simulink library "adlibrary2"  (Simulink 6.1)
undefined symbols (not defined in the file or in its folder): adlibrary2, ADM, Bit, Black, Box, d2sram_config, DDR, ddr32_config, ddr32xp_config, Generation, II, Inactive, Location, Lower, SDRAM, Simulation, Subsystem, Width, xbsIndex_r3, XPL, XRC, XRM, zbt32_config, zbt64_config, zbtXRC4_config
libraries: xbsIndex_r3 x786
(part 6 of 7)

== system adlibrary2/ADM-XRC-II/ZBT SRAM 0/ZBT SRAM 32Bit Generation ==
  d : Inport  Port=1  LatchInput=off
  a : Inport  Port=2  LatchInput=off
  w : Inport  Port=3  LatchInput=off
  r : Inport  Port=4  LatchInput=off
  be : Inport  Port=5  LatchInput=off
  adlocb_in : Inport  Port=6  LatchInput=off
  Black Box : S-Function  FunctionName=xlblackbox2  Parameters=sfcn_mwsv__  mask(Xilinx Blackbox Block){init_code=zbt32_config, sim_method=Inactive, engine_block=, show_param=on, xl_area=[88, 129, 0, 35, 0, 0, 0], xl_use_area=on, adlocb_devid=0}
      mask prompts: init_code "Block Configuration M-Function"; sim_method "Simulation Mode"; engine_block "HDL Co-Simulator To Use  (specify helper block by name)"; show_param "---------------------- Show Implementation Parameters -----------------------------------------------------------------------------------"; xl_area "FPGA Area [Slices, FFs, BRAMs, LUTs, IOBs, Emb. Mults, TBUFs]"; xl_use_area "Use Area Above For Estimation"; adlocb_devid "ADLOCB DEV ID"
      mask help: Incorporates black box HDL and simulation model into a System Generator design. You must supply a Black Box with certain information about the HDL component you would like to bring into System Generator. This information is provided through a Matlab function. When "Simulation Mode" is set to "Inactive," you will typically want to provide a separate simulation model by using a Simulation Multiplexer. When "Simulation Mode" is set to "Use HDL Co-Simulation", you must include a ModelSim block in the design.
      mask init:
      | [designRoot, family, part, speed, package, simulinkPeriod, sysclkPeriod, dbl_ovrd, trimVbit] = xlSysgenSettings(gcb,0,0);
      | 
      | [bg,fg] = xlcmap('XBlock');
      | iPos = get_param(gcb,'Position');
      | iWidth=iPos(3)-iPos(1); iHeight=iPos(4)-iPos(2);
      | iCx=iWidth/2;
      | iCy=iHeight/2;
      | [logoX, logoY] = xlogo(iPos);
      | zstr='z'; zpstr='-1';
      | zstrx = iCx-3; if (zstrx<16) zstr='';zpstr=''; end
      | zstry = iCy;
      | 
      | precision0 = 1;
      | latency = 0;
      | dblOvrd = 0;
      | 
      | mdlPath = xlGetMdlDir(bdroot);
      | 
      | refBlk = get_param(gcb,'referenceBlock');
      | if (isempty(refBlk) | strncmp(refBlk,'xbsIndex',8))
      | 	srcPath = mdlPath;
      | else
      | 	srcPath = xlPathToReference;
      | 	if (isempty(srcPath))
      | 		srcPath = mdlPath;
      | 	end
      | end
      | 
      | if (sim_method==2)
      | 	validEngineBlock = 0;
      | 	try
      | 	  engineBlock = xlBlockNameRelPath(get_param(gcb,'Parent'),engine_block);
      | 	catch
      | 	  engineBlock = '//';
      | 	end
      | 	try 
      | 	  engineWorkDir = get_param(engineBlock,'dir');
      | 	  validEngineBlock = 1;
      | 	catch
      | 	end
      | end
      | 
      | % just pass everything to s-function
      | sfcn_mwsv__ = get_param(gcb, 'MaskWSVariables');
      | 
      | plabel = xlbbPortLabelStruct(gcb,init_code,mdlPath);
  Constant : Constant  Value=0
  Convert : xbsIndex_r3/Convert  arith_type=Unsigned  n_bits=34  bin_pt=0  quantization=Truncate  overflow=Wrap  latency=0  explicit_period=on  period=1  dbl_ovrd=off  show_param=off  inserted_by_tool=off  pipeline=off
  Terminator{,1..3} (4 alike) : Terminator
  ra0 : xbsIndex_r3/Gateway Out  output_type=Double  nbits=8  bin_pt=6  arith_type=Boolean  quantization=Truncate  overflow=Wrap  hdl_port=on  timing_constraint=None  locs_specified=off  LOCs={}  needs_fixed_name=off  show_param=off
  rc0 : xbsIndex_r3/Gateway Out  output_type=Double  nbits=8  bin_pt=6  arith_type=Boolean  quantization=Truncate  overflow=Wrap  hdl_port=on  timing_constraint=None  locs_specified=off  LOCs={}  needs_fixed_name=off  show_param=off
  rd0_i : xbsIndex_r3/Gateway In  arith_type=Unsigned  n_bits=32  bin_pt=0  quantization=Truncate  overflow=Wrap  period=1  timing_constraint=None  locs_specified=off  LOCs={}  needs_fixed_name=off  dbl_ovrd=off  show_param=off
  rd0_o : xbsIndex_r3/Gateway Out  output_type=Double  nbits=8  bin_pt=6  arith_type=Boolean  quantization=Truncate  overflow=Wrap  hdl_port=on  timing_constraint=None  locs_specified=off  LOCs={}  needs_fixed_name=off  show_param=off
  rd0_t : xbsIndex_r3/Gateway Out  output_type=Double  nbits=8  bin_pt=6  arith_type=Boolean  quantization=Truncate  overflow=Wrap  hdl_port=on  timing_constraint=None  locs_specified=off  LOCs={}  needs_fixed_name=off  show_param=off
  q : Outport
  qv : Outport  Port=2
  adlocb_out : Outport  Port=3
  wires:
  Black Box/6 -> rc0/1
  Black Box/5 -> ra0/1
  Black Box/4 -> rd0_t/1
  Black Box/3 -> rd0_o/1
  r/1 -> Black Box/4
  w/1 -> Black Box/3
  a/1 -> Black Box/2
  rc0/1 -> Terminator3/1
  ra0/1 -> Terminator2/1
  rd0_t/1 -> Terminator1/1
  rd0_o/1 -> Terminator/1
  Constant/1 -> rd0_i/1
  Black Box/2 -> qv/1
  Black Box/1 -> q/1
  d/1 -> Black Box/1
  rd0_i/1 -> Black Box/6
  be/1 -> Black Box/5
  adlocb_in/1 -> Black Box/7
  Black Box/7 -> Convert/1
  Convert/1 -> adlocb_out/1

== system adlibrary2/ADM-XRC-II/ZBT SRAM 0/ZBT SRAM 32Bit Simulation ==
  d : Inport  Port=1  LatchInput=off
  a : Inport  Port=2  LatchInput=off
  w : Inport  Port=3  LatchInput=off
  r : Inport  Port=4  LatchInput=off
  be : Inport  Port=5  LatchInput=off
  Disregard Subsystem : xbsIndex_r3/Disregard Subsystem  Tag=discardX
  Gateway In6 : xbsIndex_r3/Gateway In  arith_type=Boolean  n_bits=1  bin_pt=0  quantization=Truncate  overflow=Wrap  period=1  timing_constraint=None  locs_specified=off  LOCs={}  needs_fixed_name=off  dbl_ovrd=on  show_param=off
  Gateway In7 : xbsIndex_r3/Gateway In  arith_type=Unsigned  n_bits=32  bin_pt=0  quantization=Truncate  overflow=Wrap  period=1  timing_constraint=None  locs_specified=off  LOCs={}  needs_fixed_name=off  dbl_ovrd=on  show_param=off
  Gateway Out{,1..4} (5 alike) : xbsIndex_r3/Gateway Out  output_type=Double  nbits=8  bin_pt=6  arith_type=Boolean  quantization=Truncate  overflow=Wrap  hdl_port=off  timing_constraint=None  locs_specified=off  LOCs={}  needs_fixed_name=off  show_param=off
  S-Function : S-Function  FunctionName=zbt32  Parameters=0
  q : Outport
  qv : Outport  Port=2
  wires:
  S-Function/2 -> Gateway In6/1
  Gateway In7/1 -> q/1
  Gateway In6/1 -> qv/1
  Gateway Out3/1 -> S-Function/4
  Gateway Out2/1 -> S-Function/3
  Gateway Out1/1 -> S-Function/2
  Gateway Out/1 -> S-Function/1
  S-Function/1 -> Gateway In7/1
  r/1 -> Gateway Out3/1
  w/1 -> Gateway Out2/1
  a/1 -> Gateway Out1/1
  d/1 -> Gateway Out/1
  Gateway Out4/1 -> S-Function/5
  be/1 -> Gateway Out4/1

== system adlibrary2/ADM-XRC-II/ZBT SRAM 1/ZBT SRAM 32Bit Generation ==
  d : Inport  Port=1  LatchInput=off
  a : Inport  Port=2  LatchInput=off
  w : Inport  Port=3  LatchInput=off
  r : Inport  Port=4  LatchInput=off
  be : Inport  Port=5  LatchInput=off
  adlocb_in : Inport  Port=6  LatchInput=off
  Black Box : S-Function  FunctionName=xlblackbox2  Parameters=sfcn_mwsv__  mask(Xilinx Blackbox Block){init_code=zbt32_config, sim_method=Inactive, engine_block=, show_param=on, xl_area=[88, 129, 0, 35, 0, 0, 0], xl_use_area=on, adlocb_devid=1}
      mask prompts: init_code "Block Configuration M-Function"; sim_method "Simulation Mode"; engine_block "HDL Co-Simulator To Use  (specify helper block by name)"; show_param "---------------------- Show Implementation Parameters -----------------------------------------------------------------------------------"; xl_area "FPGA Area [Slices, FFs, BRAMs, LUTs, IOBs, Emb. Mults, TBUFs]"; xl_use_area "Use Area Above For Estimation"; adlocb_devid "ADLOCB DEV ID"
      mask help: Incorporates black box HDL and simulation model into a System Generator design. You must supply a Black Box with certain information about the HDL component you would like to bring into System Generator. This information is provided through a Matlab function. When "Simulation Mode" is set to "Inactive," you will typically want to provide a separate simulation model by using a Simulation Multiplexer. When "Simulation Mode" is set to "Use HDL Co-Simulation", you must include a ModelSim block in the design.
      mask init:
      | [designRoot, family, part, speed, package, simulinkPeriod, sysclkPeriod, dbl_ovrd, trimVbit] = xlSysgenSettings(gcb,0,0);
      | 
      | [bg,fg] = xlcmap('XBlock');
      | iPos = get_param(gcb,'Position');
      | iWidth=iPos(3)-iPos(1); iHeight=iPos(4)-iPos(2);
      | iCx=iWidth/2;
      | iCy=iHeight/2;
      | [logoX, logoY] = xlogo(iPos);
      | zstr='z'; zpstr='-1';
      | zstrx = iCx-3; if (zstrx<16) zstr='';zpstr=''; end
      | zstry = iCy;
      | 
      | precision0 = 1;
      | latency = 0;
      | dblOvrd = 0;
      | 
      | mdlPath = xlGetMdlDir(bdroot);
      | 
      | refBlk = get_param(gcb,'referenceBlock');
      | if (isempty(refBlk) | strncmp(refBlk,'xbsIndex',8))
      | 	srcPath = mdlPath;
      | else
      | 	srcPath = xlPathToReference;
      | 	if (isempty(srcPath))
      | 		srcPath = mdlPath;
      | 	end
      | end
      | 
      | if (sim_method==2)
      | 	validEngineBlock = 0;
      | 	try
      | 	  engineBlock = xlBlockNameRelPath(get_param(gcb,'Parent'),engine_block);
      | 	catch
      | 	  engineBlock = '//';
      | 	end
      | 	try 
      | 	  engineWorkDir = get_param(engineBlock,'dir');
      | 	  validEngineBlock = 1;
      | 	catch
      | 	end
      | end
      | 
      | % just pass everything to s-function
      | sfcn_mwsv__ = get_param(gcb, 'MaskWSVariables');
      | adlocb_devid = 1;
      | plabel = xlbbPortLabelStruct(gcb,init_code,mdlPath);
  Constant : Constant  Value=0
  Terminator{,1..3} (4 alike) : Terminator
  ra1 : xbsIndex_r3/Gateway Out  output_type=Double  nbits=8  bin_pt=6  arith_type=Boolean  quantization=Truncate  overflow=Wrap  hdl_port=on  timing_constraint=None  locs_specified=off  LOCs={}  needs_fixed_name=off  show_param=off
  rc1 : xbsIndex_r3/Gateway Out  output_type=Double  nbits=8  bin_pt=6  arith_type=Boolean  quantization=Truncate  overflow=Wrap  hdl_port=on  timing_constraint=None  locs_specified=off  LOCs={}  needs_fixed_name=off  show_param=off
  rd1_i : xbsIndex_r3/Gateway In  arith_type=Unsigned  n_bits=32  bin_pt=0  quantization=Truncate  overflow=Wrap  period=1  timing_constraint=None  locs_specified=off  LOCs={}  needs_fixed_name=off  dbl_ovrd=off  show_param=off
  rd1_o : xbsIndex_r3/Gateway Out  output_type=Double  nbits=8  bin_pt=6  arith_type=Boolean  quantization=Truncate  overflow=Wrap  hdl_port=on  timing_constraint=None  locs_specified=off  LOCs={}  needs_fixed_name=off  show_param=off
  rd1_t : xbsIndex_r3/Gateway Out  output_type=Double  nbits=8  bin_pt=6  arith_type=Boolean  quantization=Truncate  overflow=Wrap  hdl_port=on  timing_constraint=None  locs_specified=off  LOCs={}  needs_fixed_name=off  show_param=off
  q : Outport
  qv : Outport  Port=2
  adlocb_out : Outport  Port=3
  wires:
  Black Box/7 -> adlocb_out/1
  adlocb_in/1 -> Black Box/7
  be/1 -> Black Box/5
  rd1_i/1 -> Black Box/6
  d/1 -> Black Box/1
  Black Box/1 -> q/1
  Black Box/2 -> qv/1
  Constant/1 -> rd1_i/1
  rd1_o/1 -> Terminator/1
  rd1_t/1 -> Terminator1/1
  ra1/1 -> Terminator2/1
  rc1/1 -> Terminator3/1
  a/1 -> Black Box/2
  w/1 -> Black Box/3
  r/1 -> Black Box/4
  Black Box/3 -> rd1_o/1
  Black Box/4 -> rd1_t/1
  Black Box/5 -> ra1/1
  Black Box/6 -> rc1/1

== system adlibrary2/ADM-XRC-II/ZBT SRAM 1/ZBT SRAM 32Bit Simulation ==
  d : Inport  Port=1  LatchInput=off
  a : Inport  Port=2  LatchInput=off
  w : Inport  Port=3  LatchInput=off
  r : Inport  Port=4  LatchInput=off
  be : Inport  Port=5  LatchInput=off
  Disregard Subsystem : xbsIndex_r3/Disregard Subsystem  Tag=discardX
  Gateway In6 : xbsIndex_r3/Gateway In  arith_type=Boolean  n_bits=1  bin_pt=0  quantization=Truncate  overflow=Wrap  period=1  timing_constraint=None  locs_specified=off  LOCs={}  needs_fixed_name=off  dbl_ovrd=on  show_param=off
  Gateway In7 : xbsIndex_r3/Gateway In  arith_type=Unsigned  n_bits=32  bin_pt=0  quantization=Truncate  overflow=Wrap  period=1  timing_constraint=None  locs_specified=off  LOCs={}  needs_fixed_name=off  dbl_ovrd=on  show_param=off
  Gateway Out{,1..4} (5 alike) : xbsIndex_r3/Gateway Out  output_type=Double  nbits=8  bin_pt=6  arith_type=Boolean  quantization=Truncate  overflow=Wrap  hdl_port=off  timing_constraint=None  locs_specified=off  LOCs={}  needs_fixed_name=off  show_param=off
  S-Function : S-Function  FunctionName=zbt32  Parameters=1
  q : Outport
  qv : Outport  Port=2
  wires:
  be/1 -> Gateway Out4/1
  Gateway Out4/1 -> S-Function/5
  d/1 -> Gateway Out/1
  a/1 -> Gateway Out1/1
  w/1 -> Gateway Out2/1
  r/1 -> Gateway Out3/1
  S-Function/1 -> Gateway In7/1
  Gateway Out/1 -> S-Function/1
  Gateway Out1/1 -> S-Function/2
  Gateway Out2/1 -> S-Function/3
  Gateway Out3/1 -> S-Function/4
  Gateway In6/1 -> qv/1
  Gateway In7/1 -> q/1
  S-Function/2 -> Gateway In6/1

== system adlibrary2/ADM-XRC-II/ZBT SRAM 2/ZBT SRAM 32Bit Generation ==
  d : Inport  Port=1  LatchInput=off
  a : Inport  Port=2  LatchInput=off
  w : Inport  Port=3  LatchInput=off
  r : Inport  Port=4  LatchInput=off
  be : Inport  Port=5  LatchInput=off
  adlocb_in : Inport  Port=6  LatchInput=off
  Black Box : S-Function  FunctionName=xlblackbox2  Parameters=sfcn_mwsv__  mask(Xilinx Blackbox Block){init_code=zbt32_config, sim_method=Inactive, engine_block=, show_param=on, xl_area=[88, 129, 0, 35, 0, 0, 0], xl_use_area=on, adlocb_devid=2}
      mask prompts: init_code "Block Configuration M-Function"; sim_method "Simulation Mode"; engine_block "HDL Co-Simulator To Use  (specify helper block by name)"; show_param "---------------------- Show Implementation Parameters -----------------------------------------------------------------------------------"; xl_area "FPGA Area [Slices, FFs, BRAMs, LUTs, IOBs, Emb. Mults, TBUFs]"; xl_use_area "Use Area Above For Estimation"; adlocb_devid "ADLOCB DEV ID"
      mask help: Incorporates black box HDL and simulation model into a System Generator design. You must supply a Black Box with certain information about the HDL component you would like to bring into System Generator. This information is provided through a Matlab function. When "Simulation Mode" is set to "Inactive," you will typically want to provide a separate simulation model by using a Simulation Multiplexer. When "Simulation Mode" is set to "Use HDL Co-Simulation", you must include a ModelSim block in the design.
      mask init:
      | [designRoot, family, part, speed, package, simulinkPeriod, sysclkPeriod, dbl_ovrd, trimVbit] = xlSysgenSettings(gcb,0,0);
      | 
      | [bg,fg] = xlcmap('XBlock');
      | iPos = get_param(gcb,'Position');
      | iWidth=iPos(3)-iPos(1); iHeight=iPos(4)-iPos(2);
      | iCx=iWidth/2;
      | iCy=iHeight/2;
      | [logoX, logoY] = xlogo(iPos);
      | zstr='z'; zpstr='-1';
      | zstrx = iCx-3; if (zstrx<16) zstr='';zpstr=''; end
      | zstry = iCy;
      | 
      | precision0 = 1;
      | latency = 0;
      | dblOvrd = 0;
      | 
      | mdlPath = xlGetMdlDir(bdroot);
      | 
      | refBlk = get_param(gcb,'referenceBlock');
      | if (isempty(refBlk) | strncmp(refBlk,'xbsIndex',8))
      | 	srcPath = mdlPath;
      | else
      | 	srcPath = xlPathToReference;
      | 	if (isempty(srcPath))
      | 		srcPath = mdlPath;
      | 	end
      | end
      | 
      | if (sim_method==2)
      | 	validEngineBlock = 0;
      | 	try
      | 	  engineBlock = xlBlockNameRelPath(get_param(gcb,'Parent'),engine_block);
      | 	catch
      | 	  engineBlock = '//';
      | 	end
      | 	try 
      | 	  engineWorkDir = get_param(engineBlock,'dir');
      | 	  validEngineBlock = 1;
      | 	catch
      | 	end
      | end
      | 
      | % just pass everything to s-function
      | sfcn_mwsv__ = get_param(gcb, 'MaskWSVariables');
      | 
      | plabel = xlbbPortLabelStruct(gcb,init_code,mdlPath);
  Constant : Constant  Value=0
  Terminator{,1..3} (4 alike) : Terminator
  ra2 : xbsIndex_r3/Gateway Out  output_type=Double  nbits=8  bin_pt=6  arith_type=Boolean  quantization=Truncate  overflow=Wrap  hdl_port=on  timing_constraint=None  locs_specified=off  LOCs={}  needs_fixed_name=off  show_param=off
  rc2 : xbsIndex_r3/Gateway Out  output_type=Double  nbits=8  bin_pt=6  arith_type=Boolean  quantization=Truncate  overflow=Wrap  hdl_port=on  timing_constraint=None  locs_specified=off  LOCs={}  needs_fixed_name=off  show_param=off
  rd2_i : xbsIndex_r3/Gateway In  arith_type=Unsigned  n_bits=32  bin_pt=0  quantization=Truncate  overflow=Wrap  period=1  timing_constraint=None  locs_specified=off  LOCs={}  needs_fixed_name=off  dbl_ovrd=off  show_param=off
  rd2_o : xbsIndex_r3/Gateway Out  output_type=Double  nbits=8  bin_pt=6  arith_type=Boolean  quantization=Truncate  overflow=Wrap  hdl_port=on  timing_constraint=None  locs_specified=off  LOCs={}  needs_fixed_name=off  show_param=off
  rd2_t : xbsIndex_r3/Gateway Out  output_type=Double  nbits=8  bin_pt=6  arith_type=Boolean  quantization=Truncate  overflow=Wrap  hdl_port=on  timing_constraint=None  locs_specified=off  LOCs={}  needs_fixed_name=off  show_param=off
  q : Outport
  qv : Outport  Port=2
  adlocb_out : Outport  Port=3
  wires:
  Black Box/7 -> adlocb_out/1
  adlocb_in/1 -> Black Box/7
  be/1 -> Black Box/5
  rd2_i/1 -> Black Box/6
  d/1 -> Black Box/1
  Black Box/1 -> q/1
  Black Box/2 -> qv/1
  Constant/1 -> rd2_i/1
  rd2_o/1 -> Terminator/1
  rd2_t/1 -> Terminator1/1
  ra2/1 -> Terminator2/1
  rc2/1 -> Terminator3/1
  a/1 -> Black Box/2
  w/1 -> Black Box/3
  r/1 -> Black Box/4
  Black Box/3 -> rd2_o/1
  Black Box/4 -> rd2_t/1
  Black Box/5 -> ra2/1
  Black Box/6 -> rc2/1

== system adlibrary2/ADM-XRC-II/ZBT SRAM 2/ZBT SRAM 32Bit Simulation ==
  d : Inport  Port=1  LatchInput=off
  a : Inport  Port=2  LatchInput=off
  w : Inport  Port=3  LatchInput=off
  r : Inport  Port=4  LatchInput=off
  be : Inport  Port=5  LatchInput=off
  Disregard Subsystem : xbsIndex_r3/Disregard Subsystem  Tag=discardX
  Gateway In6 : xbsIndex_r3/Gateway In  arith_type=Boolean  n_bits=1  bin_pt=0  quantization=Truncate  overflow=Wrap  period=1  timing_constraint=None  locs_specified=off  LOCs={}  needs_fixed_name=off  dbl_ovrd=on  show_param=off
  Gateway In7 : xbsIndex_r3/Gateway In  arith_type=Unsigned  n_bits=32  bin_pt=0  quantization=Truncate  overflow=Wrap  period=1  timing_constraint=None  locs_specified=off  LOCs={}  needs_fixed_name=off  dbl_ovrd=on  show_param=off
  Gateway Out{,1..4} (5 alike) : xbsIndex_r3/Gateway Out  output_type=Double  nbits=8  bin_pt=6  arith_type=Boolean  quantization=Truncate  overflow=Wrap  hdl_port=off  timing_constraint=None  locs_specified=off  LOCs={}  needs_fixed_name=off  show_param=off
  S-Function : S-Function  FunctionName=zbt32  Parameters=2
  q : Outport
  qv : Outport  Port=2
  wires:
  be/1 -> Gateway Out4/1
  Gateway Out4/1 -> S-Function/5
  d/1 -> Gateway Out/1
  a/1 -> Gateway Out1/1
  w/1 -> Gateway Out2/1
  r/1 -> Gateway Out3/1
  S-Function/1 -> Gateway In7/1
  Gateway Out/1 -> S-Function/1
  Gateway Out1/1 -> S-Function/2
  Gateway Out2/1 -> S-Function/3
  Gateway Out3/1 -> S-Function/4
  Gateway In6/1 -> qv/1
  Gateway In7/1 -> q/1
  S-Function/2 -> Gateway In6/1

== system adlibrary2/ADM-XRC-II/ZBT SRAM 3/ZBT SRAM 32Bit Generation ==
  d : Inport  Port=1  LatchInput=off
  a : Inport  Port=2  LatchInput=off
  w : Inport  Port=3  LatchInput=off
  r : Inport  Port=4  LatchInput=off
  be : Inport  Port=5  LatchInput=off
  adlocb_in : Inport  Port=6  LatchInput=off
  Black Box : S-Function  FunctionName=xlblackbox2  Parameters=sfcn_mwsv__  mask(Xilinx Blackbox Block){init_code=zbt32_config, sim_method=Inactive, engine_block=, show_param=on, xl_area=[88, 129, 0, 35, 0, 0, 0], xl_use_area=on, adlocb_devid=3}
      mask prompts: init_code "Block Configuration M-Function"; sim_method "Simulation Mode"; engine_block "HDL Co-Simulator To Use  (specify helper block by name)"; show_param "---------------------- Show Implementation Parameters -----------------------------------------------------------------------------------"; xl_area "FPGA Area [Slices, FFs, BRAMs, LUTs, IOBs, Emb. Mults, TBUFs]"; xl_use_area "Use Area Above For Estimation"; adlocb_devid "ADLOCB DEV ID"
      mask help: Incorporates black box HDL and simulation model into a System Generator design. You must supply a Black Box with certain information about the HDL component you would like to bring into System Generator. This information is provided through a Matlab function. When "Simulation Mode" is set to "Inactive," you will typically want to provide a separate simulation model by using a Simulation Multiplexer. When "Simulation Mode" is set to "Use HDL Co-Simulation", you must include a ModelSim block in the design.
      mask init:
      | [designRoot, family, part, speed, package, simulinkPeriod, sysclkPeriod, dbl_ovrd, trimVbit] = xlSysgenSettings(gcb,0,0);
      | 
      | [bg,fg] = xlcmap('XBlock');
      | iPos = get_param(gcb,'Position');
      | iWidth=iPos(3)-iPos(1); iHeight=iPos(4)-iPos(2);
      | iCx=iWidth/2;
      | iCy=iHeight/2;
      | [logoX, logoY] = xlogo(iPos);
      | zstr='z'; zpstr='-1';
      | zstrx = iCx-3; if (zstrx<16) zstr='';zpstr=''; end
      | zstry = iCy;
      | 
      | precision0 = 1;
      | latency = 0;
      | dblOvrd = 0;
      | 
      | mdlPath = xlGetMdlDir(bdroot);
      | 
      | refBlk = get_param(gcb,'referenceBlock');
      | if (isempty(refBlk) | strncmp(refBlk,'xbsIndex',8))
      | 	srcPath = mdlPath;
      | else
      | 	srcPath = xlPathToReference;
      | 	if (isempty(srcPath))
      | 		srcPath = mdlPath;
      | 	end
      | end
      | 
      | if (sim_method==2)
      | 	validEngineBlock = 0;
      | 	try
      | 	  engineBlock = xlBlockNameRelPath(get_param(gcb,'Parent'),engine_block);
      | 	catch
      | 	  engineBlock = '//';
      | 	end
      | 	try 
      | 	  engineWorkDir = get_param(engineBlock,'dir');
      | 	  validEngineBlock = 1;
      | 	catch
      | 	end
      | end
      | 
      | % just pass everything to s-function
      | sfcn_mwsv__ = get_param(gcb, 'MaskWSVariables');
      | adlocb_devid = 1;
      | plabel = xlbbPortLabelStruct(gcb,init_code,mdlPath);
  Constant : Constant  Value=0
  Terminator{,1..3} (4 alike) : Terminator
  ra3 : xbsIndex_r3/Gateway Out  output_type=Double  nbits=8  bin_pt=6  arith_type=Boolean  quantization=Truncate  overflow=Wrap  hdl_port=on  timing_constraint=None  locs_specified=off  LOCs={}  needs_fixed_name=off  show_param=off
  rc3 : xbsIndex_r3/Gateway Out  output_type=Double  nbits=8  bin_pt=6  arith_type=Boolean  quantization=Truncate  overflow=Wrap  hdl_port=on  timing_constraint=None  locs_specified=off  LOCs={}  needs_fixed_name=off  show_param=off
  rd3_i : xbsIndex_r3/Gateway In  arith_type=Unsigned  n_bits=32  bin_pt=0  quantization=Truncate  overflow=Wrap  period=1  timing_constraint=None  locs_specified=off  LOCs={}  needs_fixed_name=off  dbl_ovrd=off  show_param=off
  rd3_o : xbsIndex_r3/Gateway Out  output_type=Double  nbits=8  bin_pt=6  arith_type=Boolean  quantization=Truncate  overflow=Wrap  hdl_port=on  timing_constraint=None  locs_specified=off  LOCs={}  needs_fixed_name=off  show_param=off
  rd3_t : xbsIndex_r3/Gateway Out  output_type=Double  nbits=8  bin_pt=6  arith_type=Boolean  quantization=Truncate  overflow=Wrap  hdl_port=on  timing_constraint=None  locs_specified=off  LOCs={}  needs_fixed_name=off  show_param=off
  q : Outport
  qv : Outport  Port=2
  adlocb_out : Outport  Port=3
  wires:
  Black Box/6 -> rc3/1
  Black Box/5 -> ra3/1
  Black Box/4 -> rd3_t/1
  Black Box/3 -> rd3_o/1
  r/1 -> Black Box/4
  w/1 -> Black Box/3
  a/1 -> Black Box/2
  rc3/1 -> Terminator3/1
  ra3/1 -> Terminator2/1
  rd3_t/1 -> Terminator1/1
  rd3_o/1 -> Terminator/1
  Constant/1 -> rd3_i/1
  Black Box/2 -> qv/1
  Black Box/1 -> q/1
  d/1 -> Black Box/1
  rd3_i/1 -> Black Box/6
  be/1 -> Black Box/5
  adlocb_in/1 -> Black Box/7
  Black Box/7 -> adlocb_out/1

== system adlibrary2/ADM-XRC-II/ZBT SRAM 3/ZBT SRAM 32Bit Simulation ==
  d : Inport  Port=1  LatchInput=off
  a : Inport  Port=2  LatchInput=off
  w : Inport  Port=3  LatchInput=off
  r : Inport  Port=4  LatchInput=off
  be : Inport  Port=5  LatchInput=off
  Disregard Subsystem : xbsIndex_r3/Disregard Subsystem  Tag=discardX
  Gateway In6 : xbsIndex_r3/Gateway In  arith_type=Boolean  n_bits=1  bin_pt=0  quantization=Truncate  overflow=Wrap  period=1  timing_constraint=None  locs_specified=off  LOCs={}  needs_fixed_name=off  dbl_ovrd=on  show_param=off
  Gateway In7 : xbsIndex_r3/Gateway In  arith_type=Unsigned  n_bits=32  bin_pt=0  quantization=Truncate  overflow=Wrap  period=1  timing_constraint=None  locs_specified=off  LOCs={}  needs_fixed_name=off  dbl_ovrd=on  show_param=off
  Gateway Out{,1..4} (5 alike) : xbsIndex_r3/Gateway Out  output_type=Double  nbits=8  bin_pt=6  arith_type=Boolean  quantization=Truncate  overflow=Wrap  hdl_port=off  timing_constraint=None  locs_specified=off  LOCs={}  needs_fixed_name=off  show_param=off
  S-Function : S-Function  FunctionName=zbt32  Parameters=3
  q : Outport
  qv : Outport  Port=2
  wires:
  S-Function/2 -> Gateway In6/1
  Gateway In7/1 -> q/1
  Gateway In6/1 -> qv/1
  Gateway Out3/1 -> S-Function/4
  Gateway Out2/1 -> S-Function/3
  Gateway Out1/1 -> S-Function/2
  Gateway Out/1 -> S-Function/1
  S-Function/1 -> Gateway In7/1
  r/1 -> Gateway Out3/1
  w/1 -> Gateway Out2/1
  a/1 -> Gateway Out1/1
  d/1 -> Gateway Out/1
  Gateway Out4/1 -> S-Function/5
  be/1 -> Gateway Out4/1

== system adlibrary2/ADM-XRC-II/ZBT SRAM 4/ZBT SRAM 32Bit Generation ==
  d : Inport  Port=1  LatchInput=off
  a : Inport  Port=2  LatchInput=off
  w : Inport  Port=3  LatchInput=off
  r : Inport  Port=4  LatchInput=off
  be : Inport  Port=5  LatchInput=off
  adlocb_in : Inport  Port=6  LatchInput=off
  Black Box : S-Function  FunctionName=xlblackbox2  Parameters=sfcn_mwsv__  mask(Xilinx Blackbox Block){init_code=zbt32_config, sim_method=Inactive, engine_block=, show_param=on, xl_area=[88, 129, 0, 35, 0, 0, 0], xl_use_area=on, adlocb_devid=4}
      mask prompts: init_code "Block Configuration M-Function"; sim_method "Simulation Mode"; engine_block "HDL Co-Simulator To Use  (specify helper block by name)"; show_param "---------------------- Show Implementation Parameters -----------------------------------------------------------------------------------"; xl_area "FPGA Area [Slices, FFs, BRAMs, LUTs, IOBs, Emb. Mults, TBUFs]"; xl_use_area "Use Area Above For Estimation"; adlocb_devid "ADLOCB DEV ID"
      mask help: Incorporates black box HDL and simulation model into a System Generator design. You must supply a Black Box with certain information about the HDL component you would like to bring into System Generator. This information is provided through a Matlab function. When "Simulation Mode" is set to "Inactive," you will typically want to provide a separate simulation model by using a Simulation Multiplexer. When "Simulation Mode" is set to "Use HDL Co-Simulation", you must include a ModelSim block in the design.
      mask init:
      | [designRoot, family, part, speed, package, simulinkPeriod, sysclkPeriod, dbl_ovrd, trimVbit] = xlSysgenSettings(gcb,0,0);
      | 
      | [bg,fg] = xlcmap('XBlock');
      | iPos = get_param(gcb,'Position');
      | iWidth=iPos(3)-iPos(1); iHeight=iPos(4)-iPos(2);
      | iCx=iWidth/2;
      | iCy=iHeight/2;
      | [logoX, logoY] = xlogo(iPos);
      | zstr='z'; zpstr='-1';
      | zstrx = iCx-3; if (zstrx<16) zstr='';zpstr=''; end
      | zstry = iCy;
      | 
      | precision0 = 1;
      | latency = 0;
      | dblOvrd = 0;
      | 
      | mdlPath = xlGetMdlDir(bdroot);
      | 
      | refBlk = get_param(gcb,'referenceBlock');
      | if (isempty(refBlk) | strncmp(refBlk,'xbsIndex',8))
      | 	srcPath = mdlPath;
      | else
      | 	srcPath = xlPathToReference;
      | 	if (isempty(srcPath))
      | 		srcPath = mdlPath;
      | 	end
      | end
      | 
      | if (sim_method==2)
      | 	validEngineBlock = 0;
      | 	try
      | 	  engineBlock = xlBlockNameRelPath(get_param(gcb,'Parent'),engine_block);
      | 	catch
      | 	  engineBlock = '//';
      | 	end
      | 	try 
      | 	  engineWorkDir = get_param(engineBlock,'dir');
      | 	  validEngineBlock = 1;
      | 	catch
      | 	end
      | end
      | 
      | % just pass everything to s-function
      | sfcn_mwsv__ = get_param(gcb, 'MaskWSVariables');
      | 
      | plabel = xlbbPortLabelStruct(gcb,init_code,mdlPath);
  Constant : Constant  Value=0
  Terminator{,1..3} (4 alike) : Terminator
  ra4 : xbsIndex_r3/Gateway Out  output_type=Double  nbits=8  bin_pt=6  arith_type=Boolean  quantization=Truncate  overflow=Wrap  hdl_port=on  timing_constraint=None  locs_specified=off  LOCs={}  needs_fixed_name=off  show_param=off
  rc4 : xbsIndex_r3/Gateway Out  output_type=Double  nbits=8  bin_pt=6  arith_type=Boolean  quantization=Truncate  overflow=Wrap  hdl_port=on  timing_constraint=None  locs_specified=off  LOCs={}  needs_fixed_name=off  show_param=off
  rd4_i : xbsIndex_r3/Gateway In  arith_type=Unsigned  n_bits=32  bin_pt=0  quantization=Truncate  overflow=Wrap  period=1  timing_constraint=None  locs_specified=off  LOCs={}  needs_fixed_name=off  dbl_ovrd=off  show_param=off
  rd4_o : xbsIndex_r3/Gateway Out  output_type=Double  nbits=8  bin_pt=6  arith_type=Boolean  quantization=Truncate  overflow=Wrap  hdl_port=on  timing_constraint=None  locs_specified=off  LOCs={}  needs_fixed_name=off  show_param=off
  rd4_t : xbsIndex_r3/Gateway Out  output_type=Double  nbits=8  bin_pt=6  arith_type=Boolean  quantization=Truncate  overflow=Wrap  hdl_port=on  timing_constraint=None  locs_specified=off  LOCs={}  needs_fixed_name=off  show_param=off
  q : Outport
  qv : Outport  Port=2
  adlocb_out : Outport  Port=3
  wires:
  Black Box/7 -> adlocb_out/1
  adlocb_in/1 -> Black Box/7
  be/1 -> Black Box/5
  rd4_i/1 -> Black Box/6
  d/1 -> Black Box/1
  Black Box/1 -> q/1
  Black Box/2 -> qv/1
  Constant/1 -> rd4_i/1
  rd4_o/1 -> Terminator/1
  rd4_t/1 -> Terminator1/1
  ra4/1 -> Terminator2/1
  rc4/1 -> Terminator3/1
  a/1 -> Black Box/2
  w/1 -> Black Box/3
  r/1 -> Black Box/4
  Black Box/3 -> rd4_o/1
  Black Box/4 -> rd4_t/1
  Black Box/5 -> ra4/1
  Black Box/6 -> rc4/1

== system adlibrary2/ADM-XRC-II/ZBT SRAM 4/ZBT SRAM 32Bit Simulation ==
  d : Inport  Port=1  LatchInput=off
  a : Inport  Port=2  LatchInput=off
  w : Inport  Port=3  LatchInput=off
  r : Inport  Port=4  LatchInput=off
  be : Inport  Port=5  LatchInput=off
  Disregard Subsystem : xbsIndex_r3/Disregard Subsystem  Tag=discardX
  Gateway In6 : xbsIndex_r3/Gateway In  arith_type=Boolean  n_bits=1  bin_pt=0  quantization=Truncate  overflow=Wrap  period=1  timing_constraint=None  locs_specified=off  LOCs={}  needs_fixed_name=off  dbl_ovrd=on  show_param=off
  Gateway In7 : xbsIndex_r3/Gateway In  arith_type=Unsigned  n_bits=32  bin_pt=0  quantization=Truncate  overflow=Wrap  period=1  timing_constraint=None  locs_specified=off  LOCs={}  needs_fixed_name=off  dbl_ovrd=on  show_param=off
  Gateway Out{,1..4} (5 alike) : xbsIndex_r3/Gateway Out  output_type=Double  nbits=8  bin_pt=6  arith_type=Boolean  quantization=Truncate  overflow=Wrap  hdl_port=off  timing_constraint=None  locs_specified=off  LOCs={}  needs_fixed_name=off  show_param=off
  S-Function : S-Function  FunctionName=zbt32  Parameters=4
  q : Outport
  qv : Outport  Port=2
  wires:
  be/1 -> Gateway Out4/1
  Gateway Out4/1 -> S-Function/5
  d/1 -> Gateway Out/1
  a/1 -> Gateway Out1/1
  w/1 -> Gateway Out2/1
  r/1 -> Gateway Out3/1
  S-Function/1 -> Gateway In7/1
  Gateway Out/1 -> S-Function/1
  Gateway Out1/1 -> S-Function/2
  Gateway Out2/1 -> S-Function/3
  Gateway Out3/1 -> S-Function/4
  Gateway In6/1 -> qv/1
  Gateway In7/1 -> q/1
  S-Function/2 -> Gateway In6/1

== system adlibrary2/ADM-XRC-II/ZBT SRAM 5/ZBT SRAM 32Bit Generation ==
  d : Inport  Port=1  LatchInput=off
  a : Inport  Port=2  LatchInput=off
  w : Inport  Port=3  LatchInput=off
  r : Inport  Port=4  LatchInput=off
  be : Inport  Port=5  LatchInput=off
  adlocb_in : Inport  Port=6  LatchInput=off
  Black Box : S-Function  FunctionName=xlblackbox2  Parameters=sfcn_mwsv__  mask(Xilinx Blackbox Block){init_code=zbt32_config, sim_method=Inactive, engine_block=, show_param=on, xl_area=[88, 129, 0, 35, 0, 0, 0], xl_use_area=on, adlocb_devid=5}
      mask prompts: init_code "Block Configuration M-Function"; sim_method "Simulation Mode"; engine_block "HDL Co-Simulator To Use  (specify helper block by name)"; show_param "---------------------- Show Implementation Parameters -----------------------------------------------------------------------------------"; xl_area "FPGA Area [Slices, FFs, BRAMs, LUTs, IOBs, Emb. Mults, TBUFs]"; xl_use_area "Use Area Above For Estimation"; adlocb_devid "ADLOCB DEV ID"
      mask help: Incorporates black box HDL and simulation model into a System Generator design. You must supply a Black Box with certain information about the HDL component you would like to bring into System Generator. This information is provided through a Matlab function. When "Simulation Mode" is set to "Inactive," you will typically want to provide a separate simulation model by using a Simulation Multiplexer. When "Simulation Mode" is set to "Use HDL Co-Simulation", you must include a ModelSim block in the design.
      mask init:
      | [designRoot, family, part, speed, package, simulinkPeriod, sysclkPeriod, dbl_ovrd, trimVbit] = xlSysgenSettings(gcb,0,0);
      | 
      | [bg,fg] = xlcmap('XBlock');
      | iPos = get_param(gcb,'Position');
      | iWidth=iPos(3)-iPos(1); iHeight=iPos(4)-iPos(2);
      | iCx=iWidth/2;
      | iCy=iHeight/2;
      | [logoX, logoY] = xlogo(iPos);
      | zstr='z'; zpstr='-1';
      | zstrx = iCx-3; if (zstrx<16) zstr='';zpstr=''; end
      | zstry = iCy;
      | 
      | precision0 = 1;
      | latency = 0;
      | dblOvrd = 0;
      | 
      | mdlPath = xlGetMdlDir(bdroot);
      | 
      | refBlk = get_param(gcb,'referenceBlock');
      | if (isempty(refBlk) | strncmp(refBlk,'xbsIndex',8))
      | 	srcPath = mdlPath;
      | else
      | 	srcPath = xlPathToReference;
      | 	if (isempty(srcPath))
      | 		srcPath = mdlPath;
      | 	end
      | end
      | 
      | if (sim_method==2)
      | 	validEngineBlock = 0;
      | 	try
      | 	  engineBlock = xlBlockNameRelPath(get_param(gcb,'Parent'),engine_block);
      | 	catch
      | 	  engineBlock = '//';
      | 	end
      | 	try 
      | 	  engineWorkDir = get_param(engineBlock,'dir');
      | 	  validEngineBlock = 1;
      | 	catch
      | 	end
      | end
      | 
      | % just pass everything to s-function
      | sfcn_mwsv__ = get_param(gcb, 'MaskWSVariables');
      | adlocb_devid = 1;
      | plabel = xlbbPortLabelStruct(gcb,init_code,mdlPath);
  Constant : Constant  Value=0
  Terminator{,1..3} (4 alike) : Terminator
  ra5 : xbsIndex_r3/Gateway Out  output_type=Double  nbits=8  bin_pt=6  arith_type=Boolean  quantization=Truncate  overflow=Wrap  hdl_port=on  timing_constraint=None  locs_specified=off  LOCs={}  needs_fixed_name=off  show_param=off
  rc5 : xbsIndex_r3/Gateway Out  output_type=Double  nbits=8  bin_pt=6  arith_type=Boolean  quantization=Truncate  overflow=Wrap  hdl_port=on  timing_constraint=None  locs_specified=off  LOCs={}  needs_fixed_name=off  show_param=off
  rd5_i : xbsIndex_r3/Gateway In  arith_type=Unsigned  n_bits=32  bin_pt=0  quantization=Truncate  overflow=Wrap  period=1  timing_constraint=None  locs_specified=off  LOCs={}  needs_fixed_name=off  dbl_ovrd=off  show_param=off
  rd5_o : xbsIndex_r3/Gateway Out  output_type=Double  nbits=8  bin_pt=6  arith_type=Boolean  quantization=Truncate  overflow=Wrap  hdl_port=on  timing_constraint=None  locs_specified=off  LOCs={}  needs_fixed_name=off  show_param=off
  rd5_t : xbsIndex_r3/Gateway Out  output_type=Double  nbits=8  bin_pt=6  arith_type=Boolean  quantization=Truncate  overflow=Wrap  hdl_port=on  timing_constraint=None  locs_specified=off  LOCs={}  needs_fixed_name=off  show_param=off
  q : Outport
  qv : Outport  Port=2
  adlocb_out : Outport  Port=3
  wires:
  Black Box/6 -> rc5/1
  Black Box/5 -> ra5/1
  Black Box/4 -> rd5_t/1
  Black Box/3 -> rd5_o/1
  r/1 -> Black Box/4
  w/1 -> Black Box/3
  a/1 -> Black Box/2
  rc5/1 -> Terminator3/1
  ra5/1 -> Terminator2/1
  rd5_t/1 -> Terminator1/1
  rd5_o/1 -> Terminator/1
  Constant/1 -> rd5_i/1
  Black Box/2 -> qv/1
  Black Box/1 -> q/1
  d/1 -> Black Box/1
  rd5_i/1 -> Black Box/6
  be/1 -> Black Box/5
  adlocb_in/1 -> Black Box/7
  Black Box/7 -> adlocb_out/1

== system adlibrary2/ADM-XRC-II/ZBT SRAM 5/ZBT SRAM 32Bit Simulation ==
  d : Inport  Port=1  LatchInput=off
  a : Inport  Port=2  LatchInput=off
  w : Inport  Port=3  LatchInput=off
  r : Inport  Port=4  LatchInput=off
  be : Inport  Port=5  LatchInput=off
  Disregard Subsystem : xbsIndex_r3/Disregard Subsystem  Tag=discardX
  Gateway In6 : xbsIndex_r3/Gateway In  arith_type=Boolean  n_bits=1  bin_pt=0  quantization=Truncate  overflow=Wrap  period=1  timing_constraint=None  locs_specified=off  LOCs={}  needs_fixed_name=off  dbl_ovrd=on  show_param=off
  Gateway In7 : xbsIndex_r3/Gateway In  arith_type=Unsigned  n_bits=32  bin_pt=0  quantization=Truncate  overflow=Wrap  period=1  timing_constraint=None  locs_specified=off  LOCs={}  needs_fixed_name=off  dbl_ovrd=on  show_param=off
  Gateway Out{,1..4} (5 alike) : xbsIndex_r3/Gateway Out  output_type=Double  nbits=8  bin_pt=6  arith_type=Boolean  quantization=Truncate  overflow=Wrap  hdl_port=off  timing_constraint=None  locs_specified=off  LOCs={}  needs_fixed_name=off  show_param=off
  S-Function : S-Function  FunctionName=zbt32  Parameters=5
  q : Outport
  qv : Outport  Port=2
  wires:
  S-Function/2 -> Gateway In6/1
  Gateway In7/1 -> q/1
  Gateway In6/1 -> qv/1
  Gateway Out3/1 -> S-Function/4
  Gateway Out2/1 -> S-Function/3
  Gateway Out1/1 -> S-Function/2
  Gateway Out/1 -> S-Function/1
  S-Function/1 -> Gateway In7/1
  r/1 -> Gateway Out3/1
  w/1 -> Gateway Out2/1
  a/1 -> Gateway Out1/1
  d/1 -> Gateway Out/1
  Gateway Out4/1 -> S-Function/5
  be/1 -> Gateway Out4/1

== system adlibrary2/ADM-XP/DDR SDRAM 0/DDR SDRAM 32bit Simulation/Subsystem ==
  In1 : Inport  Port=1  LatchInput=off
  In2 : Inport  Port=2  LatchInput=off
  Disregard Subsystem : xbsIndex_r3/Disregard Subsystem  Tag=discardX
  go0 : xbsIndex_r3/Gateway In  arith_type=Unsigned  n_bits=32  bin_pt=0  quantization=Truncate  overflow=Wrap  period=1  timing_constraint=None  locs_specified=off  LOCs={}  needs_fixed_name=off  dbl_ovrd=off  show_param=off
  go1 : xbsIndex_r3/Gateway In  arith_type=Boolean  n_bits=32  bin_pt=0  quantization=Truncate  overflow=Wrap  period=1  timing_constraint=None  locs_specified=off  LOCs={}  needs_fixed_name=off  dbl_ovrd=off  show_param=off
  Out1 : Outport
  Out2 : Outport  Port=2
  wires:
  go1/1 -> Out2/1
  go0/1 -> Out1/1
  In2/1 -> go1/1
  In1/1 -> go0/1

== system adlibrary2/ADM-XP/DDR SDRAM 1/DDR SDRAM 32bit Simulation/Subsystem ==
  In1 : Inport  Port=1  LatchInput=off
  In2 : Inport  Port=2  LatchInput=off
  Disregard Subsystem : xbsIndex_r3/Disregard Subsystem  Tag=discardX
  go0 : xbsIndex_r3/Gateway In  arith_type=Unsigned  n_bits=32  bin_pt=0  quantization=Truncate  overflow=Wrap  period=1  timing_constraint=None  locs_specified=off  LOCs={}  needs_fixed_name=off  dbl_ovrd=off  show_param=off
  go1 : xbsIndex_r3/Gateway In  arith_type=Boolean  n_bits=32  bin_pt=0  quantization=Truncate  overflow=Wrap  period=1  timing_constraint=None  locs_specified=off  LOCs={}  needs_fixed_name=off  dbl_ovrd=off  show_param=off
  Out1 : Outport
  Out2 : Outport  Port=2
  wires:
  In1/1 -> go0/1
  In2/1 -> go1/1
  go0/1 -> Out1/1
  go1/1 -> Out2/1

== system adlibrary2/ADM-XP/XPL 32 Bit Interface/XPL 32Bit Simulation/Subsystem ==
  In1 : Inport  Port=1  LatchInput=off
  In2 : Inport  Port=2  LatchInput=off
  In9 : Inport  Port=3  LatchInput=off
  In3 : Inport  Port=4  LatchInput=off
  In4 : Inport  Port=5  LatchInput=off
  In5 : Inport  Port=6  LatchInput=off
  In6 : Inport  Port=7  LatchInput=off
  In7 : Inport  Port=8  LatchInput=off
  In8 : Inport  Port=9  LatchInput=off
  Disregard Subsystem : xbsIndex_r3/Disregard Subsystem  Tag=discardX
  Gateway In{,1,4..5} (4 alike) : xbsIndex_r3/Gateway In  arith_type=Boolean  n_bits=8  bin_pt=6  quantization=Truncate  overflow=Wrap  period=1  timing_constraint=None  locs_specified=off  LOCs={}  needs_fixed_name=off  dbl_ovrd=off  show_param=off
  Gateway In2 : xbsIndex_r3/Gateway In  arith_type=Unsigned  n_bits=32  bin_pt=0  quantization=Truncate  overflow=Wrap  period=1  timing_constraint=None  locs_specified=off  LOCs={}  needs_fixed_name=off  dbl_ovrd=off  show_param=off
  Gateway In3 : xbsIndex_r3/Gateway In  arith_type=Unsigned  n_bits=32  bin_pt=0  quantization=Truncate  overflow=Wrap  period=1  timing_constraint=None  locs_specified=off  LOCs={}  needs_fixed_name=off  dbl_ovrd=off  show_param=off
  Gateway In6 : xbsIndex_r3/Gateway In  arith_type=Unsigned  n_bits=16  bin_pt=0  quantization=Truncate  overflow=Wrap  period=1  timing_constraint=None  locs_specified=off  LOCs={}  needs_fixed_name=off  dbl_ovrd=off  show_param=off
  Gateway In7 : xbsIndex_r3/Gateway In  arith_type=Unsigned  n_bits=32  bin_pt=0  quantization=Truncate  overflow=Wrap  period=1  timing_constraint=None  locs_specified=off  LOCs={}  needs_fixed_name=off  dbl_ovrd=off  show_param=off
  Gateway In8 : xbsIndex_r3/Gateway In  arith_type=Unsigned  n_bits=4  bin_pt=0  quantization=Truncate  overflow=Wrap  period=1  timing_constraint=None  locs_specified=off  LOCs={}  needs_fixed_name=off  dbl_ovrd=off  show_param=off
  Out1 : Outport
  Out2 : Outport  Port=2
  Out9 : Outport  Port=3
  Out3 : Outport  Port=4
  Out4 : Outport  Port=5
  Out5 : Outport  Port=6
  Out6 : Outport  Port=7
  Out7 : Outport  Port=8
  Out8 : Outport  Port=9
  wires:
  In1/1 -> Gateway In7/1
  In2/1 -> Gateway In6/1
  In3/1 -> Gateway In5/1
  In4/1 -> Gateway In4/1
  In5/1 -> Gateway In3/1
  In6/1 -> Gateway In2/1
  In7/1 -> Gateway In1/1
  In8/1 -> Gateway In/1
  Gateway In/1 -> Out8/1
  Gateway In1/1 -> Out7/1
  Gateway In2/1 -> Out6/1
  Gateway In3/1 -> Out5/1
  Gateway In4/1 -> Out4/1
  Gateway In5/1 -> Out3/1
  Gateway In6/1 -> Out2/1
  Gateway In7/1 -> Out1/1
  In9/1 -> Gateway In8/1
  Gateway In8/1 -> Out9/1

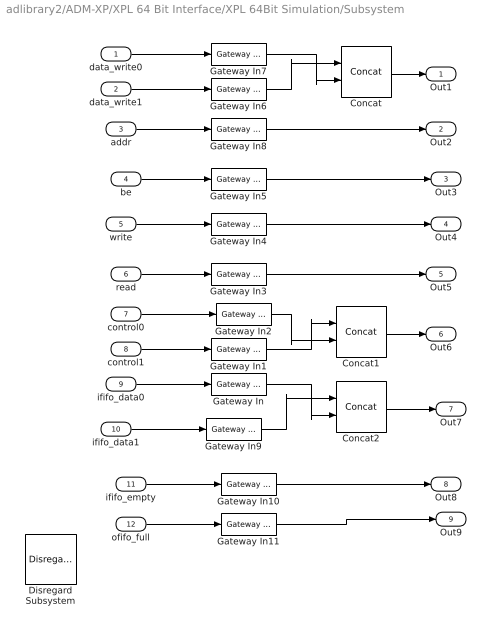
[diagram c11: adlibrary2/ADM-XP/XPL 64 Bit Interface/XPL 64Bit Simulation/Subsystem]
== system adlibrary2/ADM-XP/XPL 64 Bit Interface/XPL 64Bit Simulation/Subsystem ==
  data_write0 : Inport  Port=1  LatchInput=off
  data_write1 : Inport  Port=2  LatchInput=off
  addr : Inport  Port=3  LatchInput=off
  be : Inport  Port=4  LatchInput=off
  write : Inport  Port=5  LatchInput=off
  read : Inport  Port=6  LatchInput=off
  control0 : Inport  Port=7  LatchInput=off
  control1 : Inport  Port=8  LatchInput=off
  ififo_data0 : Inport  Port=9  LatchInput=off
  ififo_data1 : Inport  Port=10  LatchInput=off
  ififo_empty : Inport  Port=11  LatchInput=off
  ofifo_full : Inport  Port=12  LatchInput=off
  Concat : xbsIndex_r3/Concat  num_inputs=2  explicit_period=off  period=1  dbl_ovrd=off
  Concat1 : xbsIndex_r3/Concat  num_inputs=2  explicit_period=off  period=1  dbl_ovrd=off
  Concat2 : xbsIndex_r3/Concat  num_inputs=2  explicit_period=off  period=1  dbl_ovrd=off
  Disregard Subsystem : xbsIndex_r3/Disregard Subsystem  Tag=discardX
  Gateway In{,1..2,6..7,9} (6 alike) : xbsIndex_r3/Gateway In  arith_type=Unsigned  n_bits=32  bin_pt=0  quantization=Truncate  overflow=Wrap  period=1  timing_constraint=None  locs_specified=off  LOCs={}  needs_fixed_name=off  dbl_ovrd=off  show_param=off
  Gateway In10 : xbsIndex_r3/Gateway In  arith_type=Boolean  n_bits=8  bin_pt=6  quantization=Truncate  overflow=Wrap  period=1  timing_constraint=None  locs_specified=off  LOCs={}  needs_fixed_name=off  dbl_ovrd=off  show_param=off
  Gateway In11 : xbsIndex_r3/Gateway In  arith_type=Boolean  n_bits=8  bin_pt=6  quantization=Truncate  overflow=Wrap  period=1  timing_constraint=None  locs_specified=off  LOCs={}  needs_fixed_name=off  dbl_ovrd=off  show_param=off
  Gateway In3 : xbsIndex_r3/Gateway In  arith_type=Boolean  n_bits=32  bin_pt=0  quantization=Truncate  overflow=Wrap  period=1  timing_constraint=None  locs_specified=off  LOCs={}  needs_fixed_name=off  dbl_ovrd=off  show_param=off
  Gateway In4 : xbsIndex_r3/Gateway In  arith_type=Boolean  n_bits=8  bin_pt=6  quantization=Truncate  overflow=Wrap  period=1  timing_constraint=None  locs_specified=off  LOCs={}  needs_fixed_name=off  dbl_ovrd=off  show_param=off
  Gateway In5 : xbsIndex_r3/Gateway In  arith_type=Unsigned  n_bits=8  bin_pt=0  quantization=Truncate  overflow=Wrap  period=1  timing_constraint=None  locs_specified=off  LOCs={}  needs_fixed_name=off  dbl_ovrd=off  show_param=off
  Gateway In8 : xbsIndex_r3/Gateway In  arith_type=Unsigned  n_bits=16  bin_pt=0  quantization=Truncate  overflow=Wrap  period=1  timing_constraint=None  locs_specified=off  LOCs={}  needs_fixed_name=off  dbl_ovrd=off  show_param=off
  Out1 : Outport
  Out2 : Outport  Port=2
  Out3 : Outport  Port=3
  Out4 : Outport  Port=4
  Out5 : Outport  Port=5
  Out6 : Outport  Port=6
  Out7 : Outport  Port=7
  Out8 : Outport  Port=8
  Out9 : Outport  Port=9
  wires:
  Gateway In11/1 -> Out9/1
  Gateway In10/1 -> Out8/1
  Concat2/1 -> Out7/1
  Gateway In/1 -> Concat2/2
  Gateway In9/1 -> Concat2/1
  ofifo_full/1 -> Gateway In11/1
  ififo_empty/1 -> Gateway In10/1
  ififo_data1/1 -> Gateway In9/1
  Concat1/1 -> Out6/1
  Gateway In1/1 -> Concat1/1
  Gateway In2/1 -> Concat1/2
  Gateway In3/1 -> Out5/1
  Gateway In4/1 -> Out4/1
  Gateway In5/1 -> Out3/1
  Gateway In8/1 -> Out2/1
  Concat/1 -> Out1/1
  Gateway In7/1 -> Concat/2
  Gateway In6/1 -> Concat/1
  addr/1 -> Gateway In8/1
  ififo_data0/1 -> Gateway In/1
  control1/1 -> Gateway In1/1
  control0/1 -> Gateway In2/1
  read/1 -> Gateway In3/1
  write/1 -> Gateway In4/1
  be/1 -> Gateway In5/1
  data_write1/1 -> Gateway In6/1
  data_write0/1 -> Gateway In7/1

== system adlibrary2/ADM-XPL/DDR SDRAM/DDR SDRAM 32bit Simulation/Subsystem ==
  In1 : Inport  Port=1  LatchInput=off
  In2 : Inport  Port=2  LatchInput=off
  Disregard Subsystem : xbsIndex_r3/Disregard Subsystem  Tag=discardX
  go0 : xbsIndex_r3/Gateway In  arith_type=Unsigned  n_bits=32  bin_pt=0  quantization=Truncate  overflow=Wrap  period=1  timing_constraint=None  locs_specified=off  LOCs={}  needs_fixed_name=off  dbl_ovrd=off  show_param=off
  go1 : xbsIndex_r3/Gateway In  arith_type=Boolean  n_bits=32  bin_pt=0  quantization=Truncate  overflow=Wrap  period=1  timing_constraint=None  locs_specified=off  LOCs={}  needs_fixed_name=off  dbl_ovrd=off  show_param=off
  Out1 : Outport
  Out2 : Outport  Port=2
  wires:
  In1/1 -> go0/1
  In2/1 -> go1/1
  go0/1 -> Out1/1
  go1/1 -> Out2/1

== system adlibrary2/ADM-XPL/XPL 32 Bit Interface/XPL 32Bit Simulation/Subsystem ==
  In1 : Inport  Port=1  LatchInput=off
  In2 : Inport  Port=2  LatchInput=off
  In9 : Inport  Port=3  LatchInput=off
  In3 : Inport  Port=4  LatchInput=off
  In4 : Inport  Port=5  LatchInput=off
  In5 : Inport  Port=6  LatchInput=off
  In6 : Inport  Port=7  LatchInput=off
  In7 : Inport  Port=8  LatchInput=off
  In8 : Inport  Port=9  LatchInput=off
  Disregard Subsystem : xbsIndex_r3/Disregard Subsystem  Tag=discardX
  Gateway In{,1,4..5} (4 alike) : xbsIndex_r3/Gateway In  arith_type=Boolean  n_bits=8  bin_pt=6  quantization=Truncate  overflow=Wrap  period=1  timing_constraint=None  locs_specified=off  LOCs={}  needs_fixed_name=off  dbl_ovrd=off  show_param=off
  Gateway In2 : xbsIndex_r3/Gateway In  arith_type=Unsigned  n_bits=32  bin_pt=0  quantization=Truncate  overflow=Wrap  period=1  timing_constraint=None  locs_specified=off  LOCs={}  needs_fixed_name=off  dbl_ovrd=off  show_param=off
  Gateway In3 : xbsIndex_r3/Gateway In  arith_type=Unsigned  n_bits=32  bin_pt=0  quantization=Truncate  overflow=Wrap  period=1  timing_constraint=None  locs_specified=off  LOCs={}  needs_fixed_name=off  dbl_ovrd=off  show_param=off
  Gateway In6 : xbsIndex_r3/Gateway In  arith_type=Unsigned  n_bits=16  bin_pt=0  quantization=Truncate  overflow=Wrap  period=1  timing_constraint=None  locs_specified=off  LOCs={}  needs_fixed_name=off  dbl_ovrd=off  show_param=off
  Gateway In7 : xbsIndex_r3/Gateway In  arith_type=Unsigned  n_bits=32  bin_pt=0  quantization=Truncate  overflow=Wrap  period=1  timing_constraint=None  locs_specified=off  LOCs={}  needs_fixed_name=off  dbl_ovrd=off  show_param=off
  Gateway In8 : xbsIndex_r3/Gateway In  arith_type=Unsigned  n_bits=4  bin_pt=0  quantization=Truncate  overflow=Wrap  period=1  timing_constraint=None  locs_specified=off  LOCs={}  needs_fixed_name=off  dbl_ovrd=off  show_param=off
  Out1 : Outport
  Out2 : Outport  Port=2
  Out9 : Outport  Port=3
  Out3 : Outport  Port=4
  Out4 : Outport  Port=5
  Out5 : Outport  Port=6
  Out6 : Outport  Port=7
  Out7 : Outport  Port=8
  Out8 : Outport  Port=9
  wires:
  Gateway In8/1 -> Out9/1
  In9/1 -> Gateway In8/1
  Gateway In7/1 -> Out1/1
  Gateway In6/1 -> Out2/1
  Gateway In5/1 -> Out3/1
  Gateway In4/1 -> Out4/1
  Gateway In3/1 -> Out5/1
  Gateway In2/1 -> Out6/1
  Gateway In1/1 -> Out7/1
  Gateway In/1 -> Out8/1
  In8/1 -> Gateway In/1
  In7/1 -> Gateway In1/1
  In6/1 -> Gateway In2/1
  In5/1 -> Gateway In3/1
  In4/1 -> Gateway In4/1
  In3/1 -> Gateway In5/1
  In2/1 -> Gateway In6/1
  In1/1 -> Gateway In7/1
